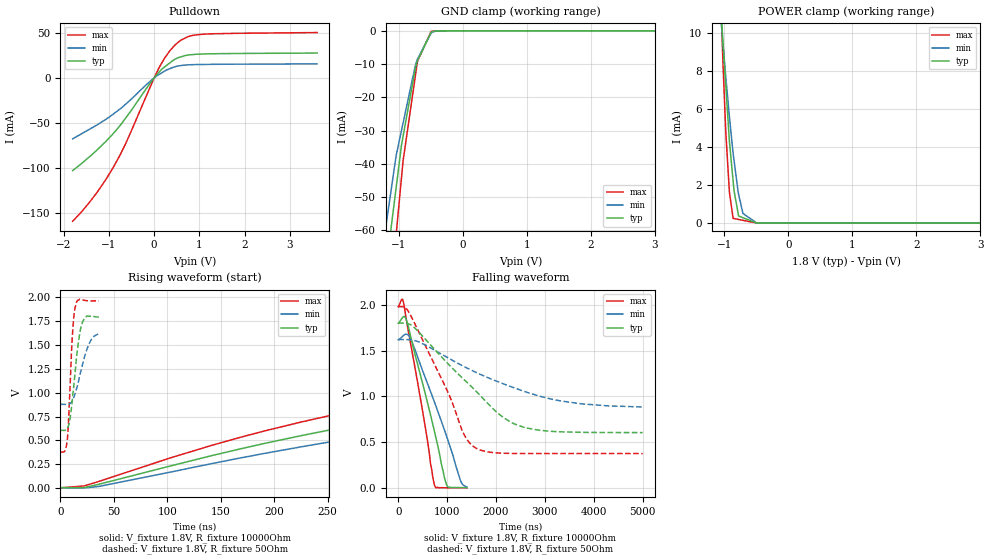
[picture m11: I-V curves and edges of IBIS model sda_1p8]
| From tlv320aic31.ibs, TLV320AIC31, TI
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|   sda_1p8 Model
[Model]   sda_1p8
Model_type   Open_drain
Polarity   Inverting
Vmeas = 0.9
Vref = 1.8
Cref = 10pF
Rref = 10000
|   typ   min   max
|   (nom PVT)   (fast PVT)   (slow PVT)
|C_comp from frequency sweep method (F=400KHz)
|C_comp   2.312e-11   2.229e-11   2.341e-11
|ON state : BUFFER OUTPUT TURNED LOW
|C_comp   4.087e-09   2.767e-09   5.586e-09
|OFF state: BUFFER IN HIGH IMPEDANCE
|C_comp   2.312e-11   2.229e-11   2.341e-11
|C_comp from LC tank measurement(L=1nH)
|Resonant Frequency(Hz)   2.030e+09   2.040e+09   2.020e+09
C_comp   6.153e-12   6.093e-12   6.214e-12
|ON state : BUFFER OUTPUT TURNED LOW
|Resonant Frequency(Hz)   1.980e+09   1.980e+09   1.980e+09
|C_comp   6.468e-12   6.468e-12   6.468e-12
|OFF state: BUFFER IN HIGH IMPEDANCE
|Resonant Frequency(Hz)   2.030e+09   2.040e+09   2.020e+09
|C_comp   6.153e-12   6.093e-12   6.214e-12
| Where nom  PVT is Nominal Process, 1.8V, 26C
|   Fast PVT is Strong Process,  1.98V, -40C
|   Slow PVT is Weak Process,   1.62V, 86C
[Voltage Range]   1.8   1.62   1.98
|Ambient Temperature   25   85   -40
|Junction Temperature
[Temperature Range]   26   86   -40
[Pullup Reference]   1.8   1.62   1.98
[Pulldown Reference]   0   0   0
[Power Clamp Reference]   1.8   1.62   1.98
[GND Clamp Reference]   0   0   0
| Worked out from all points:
|   slope of the pulldown table from 0 to 0.27 V, typ, clamps not added: 19.6 ohm
|   GND clamp passes 1 mA (typ) near -0.51 V on its own axis
|   POWER clamp passes 1 mA (typ) near -0.81 V on its own axis
|   falling waveform, V_fixture 1.8V, R_fixture 10000Ohm: 20-80 % time 496ns typ, 644ns min, 381ns max; typ from 1.8 V to 0.004 V
|   rising waveform, V_fixture 1.8V, R_fixture 10000Ohm: 20-80 % time 791ns typ, 873ns min, 710ns max; typ from 0.003 V to 1.79 V
|   falling waveform, V_fixture 1.8V, R_fixture 50Ohm: 20-80 % time 1.32us typ, 1.86us min, 799ns max; typ from 1.8 V to 0.605 V
|   rising waveform, V_fixture 1.8V, R_fixture 50Ohm: 20-80 % time 6.83ns typ, 10.6ns min, 3.95ns max; typ from 0.605 V to 1.79 V
[Pulldown]
|   Voltage   I(typ)   I(min)   I(max)
-1.8V     -103.1mA   -67.74mA   -159.5mA
-1.602V   -95.11mA   -62.05mA   -148.8mA
-1.243V   -79.27mA   -51.69mA   -126mA
-910.8mV  -62.28mA   -40.48mA   -100.2mA
-631.6mV  -44.74mA   -29.27mA   -73.31mA
-72mV     -4.794mA   -3.028mA   -8.271mA
128.7mV   7.567mA    4.489mA    13.24mA
344.5mV   16.66mA    10.3mA     30.12mA
568.3mV   23.11mA    13.67mA    41.24mA
756.4mV   25.55mA    14.56mA    46.15mA
1.109V    26.71mA    15.03mA    48.76mA
3.6V      27.76mA    15.63mA    50.5mA
[GND Clamp]
|   Voltage   I(typ)   I(min)   I(max)
-1.8V     -330.6mA   -175mA     -470.5mA
-1.202V   -71.76mA   -58.79mA   -94.27mA
-1.04V    -46.94mA   -37.39mA   -61.03mA
-957.6mV  -34.34mA   -29.93mA   -44.11mA
-932.6mV  -31.68mA   -27.67mA   -39.04mA
-745.2mV  -11.71mA   -10.72mA   -14.06mA
-712.8mV  -9.192mA   -8.64mA    -9.745mA
-704.9mV  -8.873mA   -8.35mA    -9.025mA
-495mV    -409.6uA   -657.6uA   -178.1uA
-424.4mV  -70.4uA    -146.2uA   -21.27uA
-306.2mV  -3.142uA   -7.691uA   -346.8nA
3.6V      0A         0A         0A
[POWER Clamp]
|   Voltage   I(typ)   I(min)   I(max)
-1.8V     58.58mA    42.75mA    96.1mA
-1.073V   12.51mA    11.5mA     13.37mA
-1.033V   10.12mA    9.9mA      9.534mA
-1.022V   9.52mA     9.438mA    8.427mA
-976.1mV  7.154mA    7.627mA    4.701mA
-920.7mV  4.294mA    5.584mA    1.615mA
-863.3mV  2.217mA    3.671mA    247uA
-849.6mV  1.724mA    3.318mA    237.9uA
-777.6mV  369.1uA    1.512mA    189.6uA
-709.6mV  280.2uA    505.5uA    143.9uA
-494.1mV  18.69nA    1.306uA    0A
3.6V      0A         0A         0A
[Ramp]
R_load = 10000
|   typ   min   max
dV/dt_r   1.07784/8.00774e-07   0.968537/8.91566e-07   1.18675/7.14644e-07
dV/dt_f   1.07834/4.95875e-07   0.969609/6.47669e-07   1.18694/3.81201e-07
[Falling Waveform]
V_fixture = 1.8V
V_fixture_min = 1.62V
V_fixture_max = 1.98V
R_fixture = 10000Ohm
|   Time   V(typ)   V(min)   V(max)
0s        1.8V       1.62V      1.98V
74.18ns   1.852V     1.65V      2.061V
109.3ns   1.872V     1.666V     2.026V
187ns     1.804V     1.677V     1.773V
273.7ns   1.613V     1.61V      1.518V
743.3ns   614.1mV    935.2mV    29.49mV
946.6ns   112.2mV    632.2mV    2.877mV
1.004us   21.01mV    543.5mV    2.42mV
1.273us   4.308mV    81.71mV    1.857mV
1.403us   3.508mV    11.01mV    1.799mV
[Rising Waveform]
V_fixture = 1.8V
V_fixture_min = 1.62V
V_fixture_max = 1.98V
R_fixture = 10000Ohm
|   Time   V(typ)   V(min)   V(max)
0s        2.765mV    3.978mV    1.759mV
35.68ns   38.58mV    16.28mV    68.23mV
141.5ns   339.8mV    256.1mV    447.5mV
223.9ns   546.4mV    429.6mV    688.8mV
406.6ns   893.1mV    733mV      1.077V
662ns     1.215V     1.023V     1.425V
934.2ns   1.43V      1.225V     1.649V
1.271us   1.591V     1.382V     1.807V
1.73us    1.705V     1.501V     1.909V
3.132us   1.791V     1.606V     1.975V
[Falling Waveform]
V_fixture = 1.8V
V_fixture_min = 1.62V
V_fixture_max = 1.98V
R_fixture = 50Ohm
|   Time   V(typ)   V(min)   V(max)
0s        1.8V       1.62V      1.98V
138.8ns   1.801V     1.621V     1.973V
243.3ns   1.786V     1.619V     1.896V
1.049us   1.341V     1.412V     1.008V
1.313us   1.201V     1.336V     609.7mV
1.583us   1.063V     1.265V     437.8mV
2.162us   765.9mV    1.136V     379.7mV
2.604us   651.5mV    1.05V      376.6mV
3.744us   608mV      919.5mV    376.3mV
5us       605.3mV    884.9mV    376.3mV
[Rising Waveform]
V_fixture = 1.8V
V_fixture_min = 1.62V
V_fixture_max = 1.98V
R_fixture = 50Ohm
|   Time   V(typ)   V(min)   V(max)
0s        605.2mV    877.9mV    376.3mV
4.55ns    605.7mV    877.5mV    395.6mV
6.5ns     624.8mV    877.7mV    514mV
7.8ns     663mV      880.2mV    759.8mV
10.95ns   907.6mV    912.9mV    1.555V
13.8ns    1.222V     993.8mV    1.897V
18.3ns    1.64V      1.19V      1.982V
20.9ns    1.749V     1.305V     1.974V
29.1ns    1.804V     1.562V     1.963V
35.9ns    1.793V     1.62V      1.964V
